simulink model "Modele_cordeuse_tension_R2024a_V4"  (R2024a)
settings: Solver=VariableStepAuto  StartTime=0.0  StopTime=10.0  RelTol=1e-3
libraries: fl_lib x15, nesl_utility x6, ee_lib x1, slpidlib x1

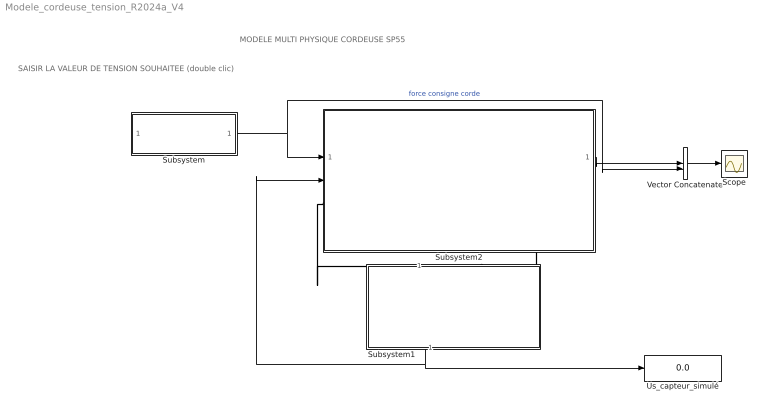
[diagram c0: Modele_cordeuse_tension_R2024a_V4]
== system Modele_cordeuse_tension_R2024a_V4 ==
  note: SAISIR LA VALEUR DE TENSION SOUHAITEE (double clic)
  note: MODELE MULTI PHYSIQUE CORDEUSE SP55
  Scope : Scope
  Subsystem : Subsystem  mask{T_kgf=4}
      mask prompts: T_kgf "Tension souhaitée (kgf)"
  Subsystem1 : Subsystem
  Subsystem2 : Subsystem
  Us_capteur_simulé : Display
  Vector Concatenate : Concatenate
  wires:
  Subsystem/1(Out1) -> Subsystem2/1(force consigne corde), Vector Concatenate/2  "force consigne corde"
  Vector Concatenate/1 -> Scope/1
  Subsystem1/1(Us_capteur_simulée) -> Us_capteur_simulé/1, Subsystem2/2(In2)
  Subsystem2/1(force effective de la corde) -> Vector Concatenate/1
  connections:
  Subsystem1/RConn1 -- Subsystem2/RConn1
  Subsystem2/LConn1 -- Subsystem1/LConn1

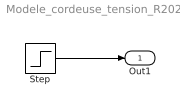
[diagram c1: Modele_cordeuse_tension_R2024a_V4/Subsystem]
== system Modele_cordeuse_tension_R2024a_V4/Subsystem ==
  Step : Step  Time=0  After=T_kgf*10  SampleTime=0
  Out1 : Outport
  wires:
  Step/1 -> Out1/1

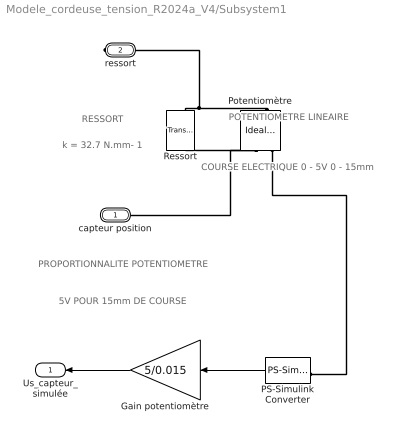
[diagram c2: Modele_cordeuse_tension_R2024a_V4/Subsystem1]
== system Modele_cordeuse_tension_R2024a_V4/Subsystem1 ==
  note: PROPORTIONNALITE POTENTIOMETRE
  note: COURSE ELECTRIQUE 0 - 5V 0 - 15mm
  note: POTENTIOMETRE LINEAIRE
  note: RESSORT
  note: k = 32.7 N.mm- 1
  note: 5V POUR 15mm DE COURSE
  Gain potentiomètre : Gain  Gain=5/0.015
  PS-Simulink Converter : nesl_utility/PS-Simulink Converter  PhysicalDomain=network_engine_domain  SubClassName=ps_output  LeftPortType=input  RightPortType=output  PseudoPeriodic=off  Frequencies=[]  VectorFormat=1-D array  Unit=1  AffineConversion=off
  Potentiomètre : fl_lib/Mechanical/Mechanical Sensors/Ideal Translational Motion Sensor  reference=foundation.enum.MeasurementReference.difference  acceleration_port=false  velocity_port=true  position_port=true  offset=0 m
  Ressort : fl_lib/Mechanical/Translational Elements/Translational Spring  spr_rate=32700 N/m  v_specify=off  v_priority=None  v=0 m/s  v_nominal_specify=off  v_nominal_value=1  v_nominal_unit=m/s  f_specify=off  f_priority=None  f=0 N  f_nominal_specify=off  f_nominal_value=1  f_nominal_unit=N  x_specify=off  x_priority=High  x=0 m  x_nominal_specify=off  x_nominal_value=1  x_nominal_unit=m
  capteur position : PMIOPort  Side=Left
  ressort : PMIOPort  Port=2  Side=Right
  Us_capteur_simulée : Outport
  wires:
  PS-Simulink Converter/1 -> Gain potentiomètre/1
  Gain potentiomètre/1 -> Us_capteur_simulée/1
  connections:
  Potentiomètre/LConn1 -- ressort/RConn1 -- Ressort/LConn1
  Potentiomètre/RConn1 -- capteur position/RConn1 -- Ressort/RConn1
  Potentiomètre/RConn3 -- PS-Simulink Converter/LConn1

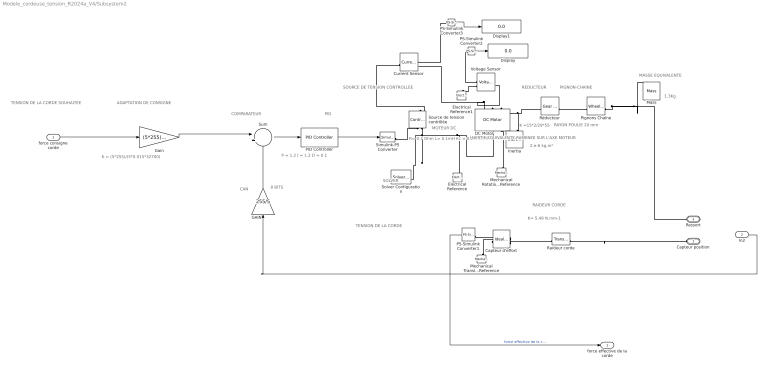
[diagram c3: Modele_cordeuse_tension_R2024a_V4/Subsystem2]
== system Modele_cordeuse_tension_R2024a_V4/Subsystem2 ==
  note: ADAPTATION DE CONSIGNE
  note: SOLVER
  note: K = (5*255)/(5*0.015*32700)
  note: SOURCE DE TENSION CONTROLLEE
  note: CAN
  note: COMPARATEUR
  note: R= 0.7 Ohm L= 0.1mH Kc = 0.03 Nm/A
  note: TENSION DE LA CORDE SOUHAITEE
  note: TENSION DE LA CORDE
  note: PID
  note: 2.e-6 kg.m²
  note: P = 1.2 I = 1.2 D = 0.1
  note: 8 BITS
  note: RAIDEUR CORDE
  note: PIGNON-CHAINE
  note: 1.3Kg
  note: MASSE EQUIVALENTE
  note: MOTEUR DC
  note: K= 5.49 N.mm-1
  note: RAYON POULIE 20 mm
  note: REDUCTEUR
  note: K =15*2/29*55
  note: I NERTIE EQUIVALENTE RAMENEE SUR L'AXE MOTEUR
  force consigne corde : Inport
  In2 : Inport  Port=2
  Capteur d'effort : fl_lib/Mechanical/Mechanical Sensors/Ideal Force Sensor
  Current Sensor : fl_lib/Electrical/Electrical Sensors/Current Sensor
  DC Motor : ee_lib/Electromechanical/Brushed Motors/DC Motor  field_option=ee.enum.field_option.pm  Rf=100 Ohm  Lf=1 H  Laf=0.15 H  If0=0 A  parameterization=1  Ra=0.7 Ohm  La=0.1 mH  emf_or_torque=2  Kv=7.2e-5 V/rpm  Ki=0.03 N*m/A  T_stall=2.4e-4 N*m  w_max=1.91e+4 rpm  w_rated=1.5e+4 rpm  P_rated=0.08 W  V_rated=1.5 V  lam_param=1  i_noload=0 A  V_i_noload=1.5 V  J=0.0001 kg*m^2  lam=0 N*m/(rad/s)  speed0=0 rpm  enable_fault_armature=simscape.enum.onoff.off  rev_faulted=1 / 3  G_faulted_armature=1e-5 S  fault_trigger_armature=ee.enum.faults.faultTrigger.temporal  t_fault_armature=1 s  max_permissible_current_armature=inf A  t_fail_on_current_armature=1 s  enable_fault_field=simscape.enum.onoff.off  G_faulted_field=1e-5 S  fault_trigger_field=ee.enum.faults.faultTrigger.temporal  t_fault_field=1 s  max_permissible_current_field=inf A  t_fail_on_current_field=1 s  fault_action=simscape.enum.assert.action.none  alpha=3.93e-3 1/K  Tmeas=25 degC  thermal_mass=100 J/K  initial_temperature=25 degC
  Display : Display
  Display1 : Display
  Electrical Reference : fl_lib/Electrical/Electrical Elements/Electrical Reference
  Electrical Reference1 : fl_lib/Electrical/Electrical Elements/Electrical Reference
  GAIN : Gain  Gain=255/5
  Gain : Gain  Gain=(5*255)/(5*0.015*32700)
  Inertia : fl_lib/Mechanical/Rotational Elements/Inertia  inertia=0.000002 kg*m^2  num_ports=foundation.enum.numPorts2.one  w_specify=off  w_priority=High  w=0 rad/s  w_nominal_specify=off  w_nominal_value=1  w_nominal_unit=rad/s  t_specify=off  t_priority=None  t=0 N*m  t_nominal_specify=off  t_nominal_value=1  t_nominal_unit=N*m
  Mass : fl_lib/Mechanical/Translational Elements/Mass  mass=1.3 kg  num_ports=foundation.enum.numPorts2.one  v_specify=off  v_priority=High  v=0 m/s  v_nominal_specify=off  v_nominal_value=1  v_nominal_unit=m/s  f_specify=off  f_priority=None  f=0 N  f_nominal_specify=off  f_nominal_value=1  f_nominal_unit=N
  Mechanical Rotational Reference : fl_lib/Mechanical/Rotational Elements/Mechanical Rotational Reference
  Mechanical Translational Reference : fl_lib/Mechanical/Translational Elements/Mechanical Translational Reference
  PID Controller : slpidlib/PID Controller  Controller=PID  Form=Parallel  TimeDomain=Continuous-time  UseExternalTs=off  SampleTime=-1  IntegratorMethod=Forward Euler  FilterMethod=Forward Euler  ControllerParametersSource=internal  P=1.2  I=1.2  UseKiTs=off  D=0.1  UseExternalDerivativeSource=off  N=100  UseFilter=on  TunerSelectOption=Transfer Function Based (PID Tuner App)  InitialConditionSource=internal  InitialConditionForIntegrator=0  InitialConditionForFilter=0  DifferentiatorICPrevScaledInput=0  ExternalReset=none  TrackingMode=off  Kt=1  LimitOutput=off  SatLimitsSource=internal  UpperSaturationLimit=inf  LowerSaturationLimit=-inf  LinearizeAsGain=on  AntiWindupMode=none  Kb=1  LimitIntegrator=off  UpperIntegratorSaturationLimit=inf  LowerIntegratorSaturationLimit=-inf  POutMin=[]  POutMax=[]  IOutMin=[]  IOutMax=[]  DOutMin=[]  DOutMax=[]  NOutMin=[]  NOutMax=[]  SumOutMin=[]  SumOutMax=[]  SaturationOutMin=[]  SaturationOutMax=[]  PParamMin=[]  PParamMax=[]  IParamMin=[]  IParamMax=[]  DParamMin=[]  DParamMax=[]  NParamMin=[]  NParamMax=[]  KbParamMin=[]  KbParamMax=[]  KtParamMin=[]  KtParamMax=[]  KbOutMin=[]  KbOutMax=[]  KtOutMin=[]  KtOutMax=[]  IntegratorOutMin=[]  IntegratorOutMax=[]  FilterOutMin=[]  FilterOutMax=[]  SumI1OutMin=[]  SumI1OutMax=[]  SumI2OutMin=[]  SumI2OutMax=[]  SumI3OutMin=[]  SumI3OutMax=[]  SumI4OutMin=[]  SumI4OutMax=[]  SumDOutMin=[]  SumDOutMax=[]  DifferentiatorOutMin=[]  DifferentiatorOutMax=[]  FilterDiffOutCoefMin=[]  FilterDiffOutCoefMax=[]  ReciprocalOutMin=[]  ReciprocalOutMax=[]  SumDenOutMin=[]  SumDenOutMax=[]  SumNumOutMin=[]  SumNumOutMax=[]  DivideOutMin=[]  DivideOutMax=[]  UdiffTsProdOutMin=[]  UdiffTsProdOutMax=[]  NTsProdOutMin=[]  NTsProdOutMax=[]  UintegralTsProdOutMin=[]  UintegralTsProdOutMax=[]  UngainTsProdOutMin=[]  UngainTsProdOutMax=[]  ClampingZeroOutDataTypeStr=Inherit: Inherit via back propagation  ClampingZeroOutMin=[]  ClampingZeroOutMax=[]  FilterDenConstantOutDataTypeStr=Inherit: Inherit via back propagation  FilterDenConstantOutMin=[]  FilterDenConstantOutMax=[]  PCopyOutDataTypeStr=Inherit: Inherit via back propagation  PCopyOutMin=[]  PCopyOutMax=[]  NCopyOutDataTypeStr=Inherit: Inherit via back propagation  NCopyOutMin=[]  NCopyOutMax=[]  IntegratorContinuousStateAttributes=''  IntegratorStateMustResolveToSignalObject=off  IntegratorRTWStateStorageClass=Auto  FilterContinuousStateAttributes=''  FilterStateMustResolveToSignalObject=off  FilterRTWStateStorageClass=Auto  ParallelPVariant=InternalParameters  IdealPVariant=Disabled  IVariant=InternalParameters  DVariant=InternalParameters  IntegratorVariant=Continuous  SatVariant=Disabled  AWVariant=Passthrough  PCopyVariant=Disabled  TRVariant=Disabled  FdbkBlocksVariant=Forward  IdealPFdbkVariant=Disabled  SatFdbkVariant=Disabled  DerivativeFilterVariant=ContFilter  NVariant=InternalParameters  NCopyVariant=Disabled  FilterICVariant=InternalICsFilter  IntegratorICVariant=InternalICs  ExternalResetVariant=Disabled  TRSumVariant=Passthrough  SumFdbkVariant=Disabled  SumVariant=Sum_PID  TsampFilterVariant=InternalTs  TsampNgainVariant=Passthrough  TsampIntegralVariant=Disabled_SignalSpec  ExternalSaturationOutDataTypeStr=Inherit: Same as second input  DerivativeSourceVariant=ErrorSignal
  PS-Simulink Converter1 : nesl_utility/PS-Simulink Converter  PhysicalDomain=network_engine_domain  SubClassName=ps_output  LeftPortType=input  RightPortType=output  PseudoPeriodic=off  Frequencies=[]  VectorFormat=1-D array  Unit=1  AffineConversion=off
  PS-Simulink Converter2 : nesl_utility/PS-Simulink Converter  PhysicalDomain=network_engine_domain  SubClassName=ps_output  LeftPortType=input  RightPortType=output  PseudoPeriodic=off  Frequencies=[]  VectorFormat=inherit  Unit=inherit  AffineConversion=off
  PS-Simulink Converter3 : nesl_utility/PS-Simulink Converter  PhysicalDomain=network_engine_domain  SubClassName=ps_output  LeftPortType=input  RightPortType=output  PseudoPeriodic=off  Frequencies=[]  VectorFormat=inherit  Unit=inherit  AffineConversion=off
  Pignons Chaîne : fl_lib/Mechanical/Mechanisms/Wheel and Axle  R=0.02 m  or=1  t_specify=off  t_priority=None  t=0 N*m  t_nominal_specify=off  t_nominal_value=1  t_nominal_unit=N*m  f_specify=off  f_priority=None  f=0 N  f_nominal_specify=off  f_nominal_value=1  f_nominal_unit=N
  Raideur corde : fl_lib/Mechanical/Translational Elements/Translational Spring  spr_rate=5490 N/m  v_specify=off  v_priority=None  v=0 m/s  v_nominal_specify=off  v_nominal_value=1  v_nominal_unit=m/s  f_specify=off  f_priority=None  f=0 N  f_nominal_specify=off  f_nominal_value=1  f_nominal_unit=N  x_specify=off  x_priority=High  x=0 m  x_nominal_specify=off  x_nominal_value=1  x_nominal_unit=m
  Réducteur : fl_lib/Mechanical/Mechanisms/Gear Box  ratio=29*55/30  t_in_specify=off  t_in_priority=None  t_in=0 N*m  t_in_nominal_specify=off  t_in_nominal_value=1  t_in_nominal_unit=N*m  t_out_specify=off  t_out_priority=None  t_out=0 N*m  t_out_nominal_specify=off  t_out_nominal_value=1  t_out_nominal_unit=N*m
  Simulink-PS Converter : nesl_utility/Simulink-PS Converter  PhysicalDomain=network_engine_domain  SubClassName=ps_input  LeftPortType=input  RightPortType=output  PseudoPeriodic=off  Frequencies=[]  NoiseDistribution=none  NoiseParameters=[]  Unit=1  AffineConversion=off  FilteringAndDerivatives=provide  SimscapeFilterOrder=1  InputFilterTimeConstant=0.001  UdotUserProvided=0
  Solver Configuration : nesl_utility/Solver Configuration  PhysicalDomain=network_engine_domain  SubClassName=solver  LeftPortType=input  RightPortType=generic  Tones=[]  Harmonics=[]  SimulateNoise=off  Profile=off  UseLocalSampling=off  EnableSwitchedLinearOptims=on  FrequencyDomain=off  UseCCode=off  RelTol=0.001  AbsTol=1e-06  MinStep=1e-09  ToWorkspace=off  RevertToSquareIcSolve=off  NumHomotopyIterations=100  PhasorMode=off  PhasorModeNumHarmonics=1  ConsistencySolver=NEWTON_FTOL  IndexReductionMethod=DerivativeReplacement  DoDC=off  ResidualTolerance=1e-09  ConsistencyTolSource=GLOBAL  ConsistencyAbsTol=0.001  ConsistencyRelTol=0.001  ConsistencyTolFactor=0.001  UseLocalSolver=off  LocalSolverChoice=NE_BACKWARD_EULER_ADVANCER  ResolveIndetEquations=on  FunctionEvalNumThread=1  LocalSolverSampleTime=0.001  DoFixedCost=off  MaxNonlinIter=3  MaxModeIter=2  ComputeImpulses=off  ImpulseIterations=2  LinearAlgebra=Sparse  LinearAlgebraNumThread=0  EquationFormulation=NE_TIME_EF  DelaysMemoryBudget=1024  AutomaticFiltering=on  FilteringTimeConstant=0.001  PartitionStorageMethod=AS_NEEDED  PartitionMemoryBudget=1024  PartitionMethod=FAST  MultibodyUseLocalSolver=off  MultibodyLocalSolverChoice=ODE1  MultibodyLocalSolverSampleTime=0.001
  Source de tension contrôlée : fl_lib/Electrical/Electrical Sources/Controlled Voltage Source
  Sum : Sum  Inputs=|+-
  Voltage Sensor : fl_lib/Electrical/Electrical Sensors/Voltage Sensor
  Capteur position : PMIOPort  Side=Left
  Ressort : PMIOPort  Port=2  Side=Right
  force effective de la corde : Outport
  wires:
  GAIN/1 -> Sum/2
  PID Controller/1 -> Simulink-PS Converter/1
  force consigne corde/1 -> Gain/1
  Gain/1 -> Sum/1
  Sum/1 -> PID Controller/1
  PS-Simulink Converter2/1 -> Display/1
  PS-Simulink Converter3/1 -> Display1/1
  PS-Simulink Converter1/1 -> force effective de la corde/1  "force effective de la corde"
  In2/1 -> GAIN/1
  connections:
  Inertia/LConn1 -- DC Motor/LConn2 -- Réducteur/LConn1
  PS-Simulink Converter3/LConn1 -- Current Sensor/RConn1
  Voltage Sensor/RConn2 -- Electrical Reference1/LConn1
  Capteur d'effort/RConn2 -- PS-Simulink Converter1/LConn1
  Pignons Chaîne/LConn1 -- Réducteur/RConn1
  Simulink-PS Converter/RConn1 -- Source de tension contrôlée/RConn1
  Mechanical Translational Reference/LConn1 -- Capteur d'effort/RConn1
  DC Motor/LConn1 -- Voltage Sensor/LConn1 -- Current Sensor/RConn2
  Source de tension contrôlée/RConn2 -- Solver Configuration/RConn1 -- Electrical Reference/LConn1 -- DC Motor/RConn1
  Pignons Chaîne/RConn1 -- Ressort/RConn1 -- Mass/LConn1
  Current Sensor/LConn1 -- Source de tension contrôlée/LConn1
  Mechanical Rotational Reference/LConn1 -- DC Motor/RConn2
  Capteur d'effort/LConn1 -- Raideur corde/RConn1
  PS-Simulink Converter2/LConn1 -- Voltage Sensor/RConn1
  Raideur corde/LConn1 -- Capteur position/RConn1
